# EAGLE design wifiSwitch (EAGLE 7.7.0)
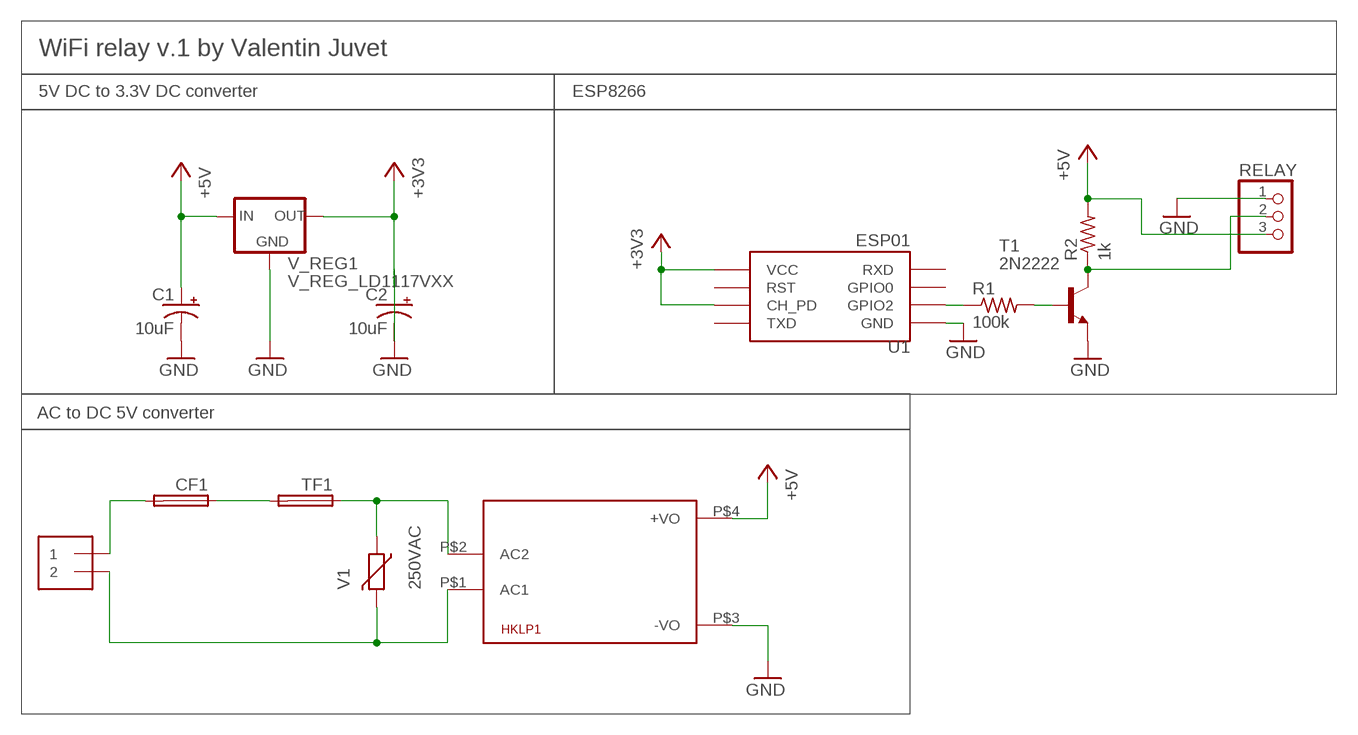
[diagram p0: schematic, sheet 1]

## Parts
C1  10uF  10UF-POLAR-RADIAL-2.5MM-25V-20%  [CPOL-RADIAL-2.5MM-5MM]
C2  10uF  10UF-POLAR-RADIAL-2.5MM-25V-20%  [CPOL-RADIAL-2.5MM-5MM]
CF1  TE5  [TE5]
HKLP1  HKLPM01  [HKLPM01]
J1  1X2-3.5MM  [1X2-3.5MM]
R1  100k  R-US_0207/10  [0207/10]
R2  1k  R-US_0207/10  [0207/10]
RELAY  PINHD-1X3CB  [1X03-CLEANBIG]
T1  2N2222  [TO92-EBC-OVAL]
TF1  TE5  [TE5]
U1  ESP01  [ESP01]
V1  250VAC  VARISTOR-7,5  [R-7,5]
V_REG1  V_REG_LD1117VXX  [78XXL]

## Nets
+3V3: C2.1(+) U1.CH_PD U1.VCC V_REG1.GND(OUT)
+5V: C1.1(+) HKLP1.P$4(+VO) R2.2 RELAY.3 V_REG1.OUT(IN)
GND: C1.2(-) C2.2(-) HKLP1.P$3(-VO) RELAY.1 T1.E U1.GND V_REG1.IN(GND)
N$1 [250AC]: CF1.2 J1.1
N$2 [250AC]: CF1.1 TF1.2
N$3 [250AC]: HKLP1.P$1(AC1) J1.2 V1.2
N$4 [250AC]: HKLP1.P$2(AC2) TF1.1 V1.1
N$5: R1.1 U1.GPIO2
N$6: R1.2 T1.B
N$7: R2.1 RELAY.2 T1.C
Unconnected: U1.GPIO0 U1.RST U1.RX(RXD) U1.TX(TXD)

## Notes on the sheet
- WiFi relay v.1 by Valentin Juvet
- 5V DC to 3.3V DC converter | ESP8266
- AC to DC 5V converter

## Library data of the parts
C1 C2 = SparkFun-Capacitors:10UF-POLAR: 10.0µF polarized capacitors; PROD_ID: CAP-08440
CF1 TF1 = fuse:TE5: FUSE; OC_FARNELL: unknown; OC_NEWARK: unknown
HKLP1 = HKLPM01:HKLPM01
J1 = adafruit:1X2: 3.5mm Terminal block
R1 R2 = adafruit:R-US_: RESISTOR, American symbol
RELAY = adafruit:PINHD-1X3: PIN HEADER
T1 = adafruit:2N2222: NPN TRANSISTOR Big oval pads
U1 = ESP8266:ESP01: ESP8266 Wifi module 01
V1 = varistor:VARISTOR: VARISTOR
V_REG1 = SparkFun-IC-Power:V_REG_LD1117VXX: LD1117VXX voltage regulator. We carry the 3.3V version (COM-00526) in TO-220 package.

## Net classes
0 default: width 0.305 mm, drill 0.508 mm, clearance 0.254 mm
1 250AC: width 1.27 mm, drill 2.032 mm, clearance 1.016 mm

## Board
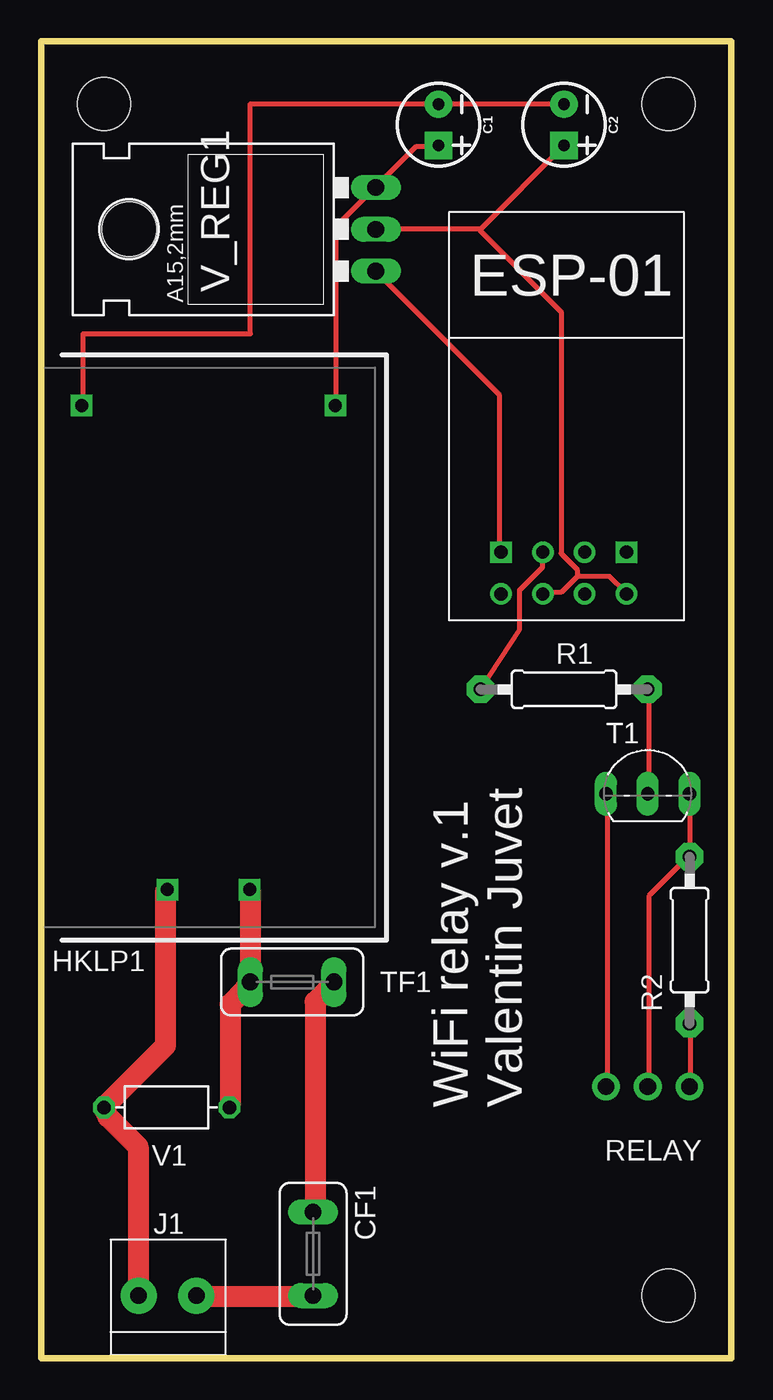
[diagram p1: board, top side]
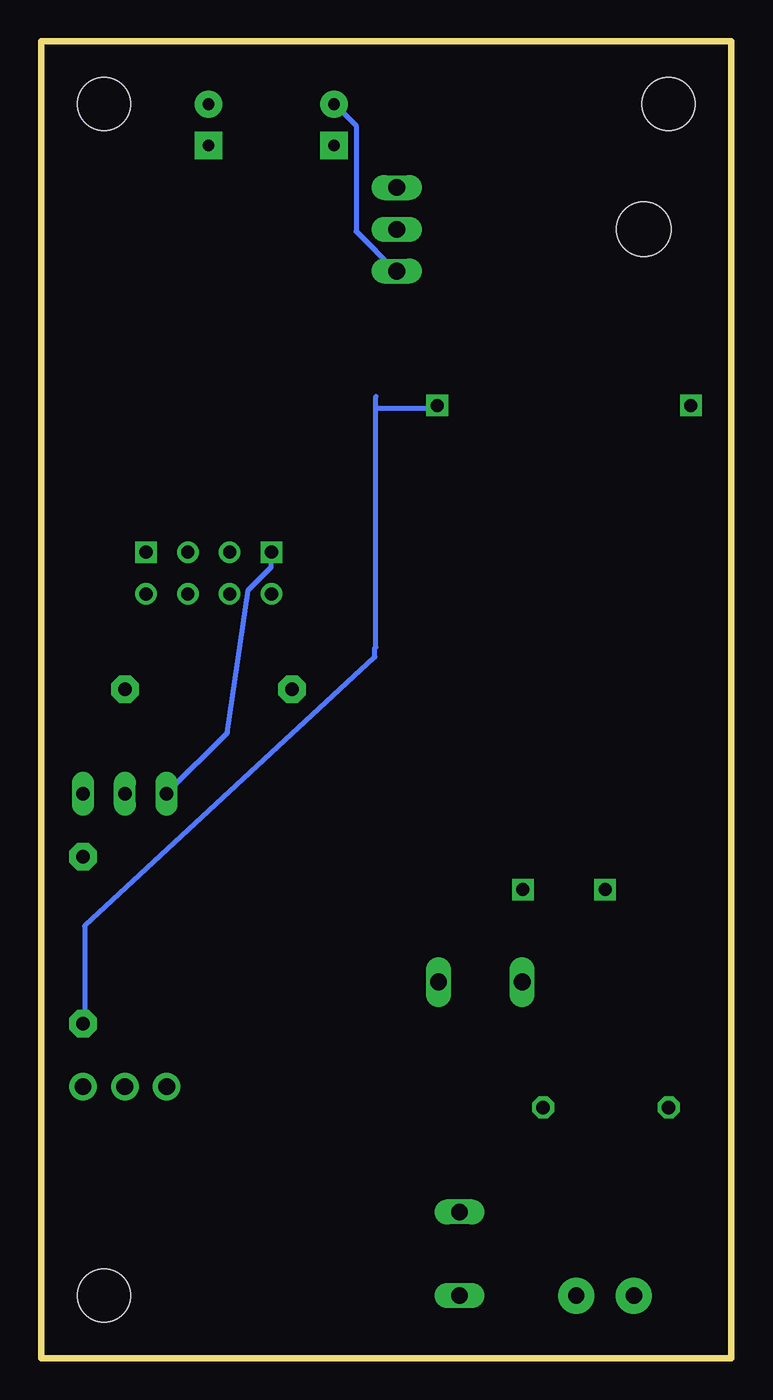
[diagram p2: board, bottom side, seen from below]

Size 41.91 x 80.01 mm. Coordinates in mm from the lower left corner, seen from the top.
Outline: 0,0 0,80.01 41.91,80.01 41.91,0 0,0
Copper layers (1*16): Top 0.035mm / dielectric 1.5mm / Bottom 0.035mm
Design rules "default": minimum track width 10mil, minimum drill 24mil, track to track 8mil, track to pad 8mil, pad to pad 8mil, via to via 8mil, smd to smd 8mil, copper to edge 40mil, drill to drill 8mil, minimum pad ring 10mil, minimum via ring 8mil, stop-mask expansion 4mil, vias tented up to drill 0mil, thermal gap 10mil
Holes 3.2 mm at 38.1,76.2 38.1,3.81 3.81,76.2

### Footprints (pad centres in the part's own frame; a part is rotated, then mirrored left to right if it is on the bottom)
CPOL-RADIAL-2.5MM-5MM = drill 0.7 pad 1.651 square: 1 1.25,0 | drill 0.7 pad 1.651: 2 -1.25,0
TE5 = drill 1.016 long: 1 -2.54,0; 2 2.54,0
HKLPM01 = drill 0.8 square: P$1 -14.7,2.5; P$2 -14.7,-2.5; P$3 14.7,7.7; P$4 14.7,-7.7
1X2-3.5MM = drill 1 pad 2.184: 1 1.8,0; 2 -1.7,0
0207/10 = drill 0.813 pad 1.676 octagon: 1 -5.08,0; 2 5.08,0
1X03-CLEANBIG = drill 1.016 pad 1.676: 1 -2.54,0; 2 0,0; 3 2.54,0
TO92-EBC-OVAL = drill 0.813 long: B 0,-1.27; C 2.54,-1.27; E -2.54,-1.27
ESP01 = drill 0.8: CH_PD -1.285,-8.178; GPIO0 1.255,-5.638; GPIO2 -1.285,-5.638; RST 1.255,-8.178; TX -3.825,-8.178; VCC 3.795,-8.178 | drill 0.8 square: GND -3.825,-5.638; RX 3.795,-5.638
R-7,5 = drill 0.813 octagon: 1 -3.81,0; 2 3.81,0
78XXL = drill 1.016 long: GND 0,-3.81; IN -2.54,-3.81; OUT 2.54,-3.81 | hole 3.302: 0,11.176

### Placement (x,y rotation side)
C1  24.13,74.93 270 top
C2  31.75,74.93 270 top
CF1  16.51,6.35 270 top
HKLP1  10.16,43.18 90 top
J1  7.62,3.81 0 top
R1  31.75,40.64 0 top
R2  39.37,25.4 270 top
RELAY  36.83,16.51 0 top
T1  36.83,35.56 0 top
TF1  15.24,22.86 0 top
U1  31.75,54.61 0 top
V1  7.62,15.24 180 top
V_REG1  16.51,68.58 90 top

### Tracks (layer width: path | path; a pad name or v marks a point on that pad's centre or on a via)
+3V3
  Top 0.305: 32.55,47.5 31.57,46.52 30.59,46.52 U1.CH_PD | 32.55,47.5 34.51,47.5 35.48,46.52 U1.VCC | 26.68,68.59 20.4,68.59 V_REG1.GND | 26.68,68.59 31.71,73.62 C2.1 | 32.55,47.5 32.55,47.92 31.57,48.9 31.57,63.56 26.68,68.45 26.68,68.59
+5V
  Top 0.305: HKLP1.P$4 17.89,57.98 17.89,68.73 20.27,71.11 V_REG1.OUT 20.41,71.25 22.78,73.62 24.04,73.62 C1.1 | RELAY.3 39.41,16.62 39.41,20.26 R2.2
  Bottom 0.305: 17.89,57.84 HKLP1.P$4 | R2.2 39.27,20.4 39.27,26.26 21.69,42.57 21.65,42.61 21.65,43.17 21.59,43.18 21.59,57.7 | 17.88,57.7 HKLP1.P$4 | 21.59,57.7 21.59,58.42 | 21.59,57.7 18.02,57.7 HKLP1.P$4
GND
  Top 0.305: RELAY.1 34.38,16.62 34.38,34.23 T1.E | U1.GND 27.8,49.03 27.8,58.53 20.4,65.94 V_REG1.IN | HKLP1.P$3 2.54,57.88 2.54,62.23 12.7,62.23 12.7,76.2 24.13,76.2 | 24.13,76.2 C1.2 | 24.13,76.2 31.75,76.2 C2.2
  Bottom 0.305: V_REG1.IN 20.41,66.08 22.78,68.45 22.78,74.88 24.04,76.14 C1.2 | U1.GND 27.94,48.9 27.94,48.06 29.34,46.66 30.61,38 34.24,34.37 T1.E
N$1
  Top 1.27: CF1.2 16.5,3.77 9.51,3.77 J1.1
N$2
  Top 1.27: CF1.1 16.64,8.94 16.64,21.65 17.75,22.77 TF1.2
N$3
  Top 1.27: HKLP1.P$1 7.56,28.36 7.56,19 3.92,15.37 V1.2 4.06,14.67 5.88,12.85 5.88,3.91 J1.2
N$4
  Top 1.27: HKLP1.P$2 12.72,28.36 12.72,22.91 TF1.1 12.31,22.35 11.47,21.51 11.47,15.37 V1.1
N$5
  Top 0.305: U1.GPIO2 30.45,48.9 30.45,48.06 29.06,46.66 29.06,44.28 26.7,40.65 R1.1
N$6
  Top 0.305: T1.B 36.89,34.37 36.89,40.51 R1.2
N$7
  Top 0.305: T1.C 39.41,34.23 39.41,30.59 R2.1 39.27,30.45 36.89,28.08 36.89,16.62 RELAY.2

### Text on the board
tNames: WiFi relay v.1 / Valentin Juvet

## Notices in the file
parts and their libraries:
SparkFun-IC-Power: Licensing: Creative Commons ShareAlike 4.0 International - https://creativecommons.org/licenses/by-sa/4.0
